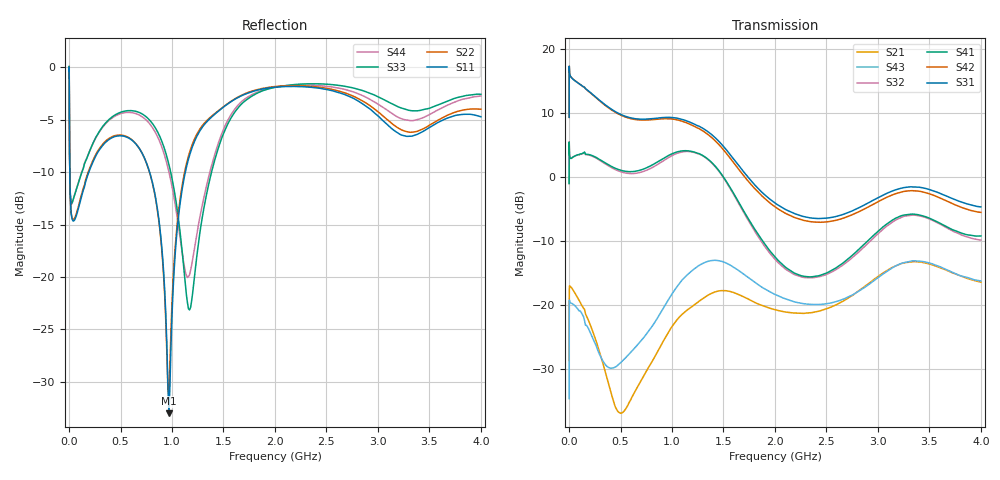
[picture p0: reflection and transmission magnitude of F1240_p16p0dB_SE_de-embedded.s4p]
! Integrated Device Technology
! Corporate Headquarters
! 6024 Silver Creek Valley Road
! San Jose, CA 95138  USA
! Phone:  1-408-284-8200
! Toll Free:  1-800-223-1366
! Webpage:  http://www.idt.com/
! Timing and RF Division
! 515 Groton Road, Suite 102
! Westford, MA 01886-6024
! Device:  F1240
! Description: Dual Intermediate Frequency Digital Variable Gain Amplifier
! Frequency:  10.0 -  500.00 MHz
! Package:  5x5 mm QFN Plastic Package: 32 pin
! Ports:  8 RF, 20 DC
!  Pin  1  = GA3 / Data  Pin 17  = RF OUT_B+
!  Pin  2  = GA4 / CLK  Pin 18  = RF OUT_B-
!  Pin  3  = GA5  Pin 19  = STBY_B
!  Pin  4  = VMODE  Pin 20  = Ground
!  Pin  5  = No Connect  Pin 21  = Ground
!  Pin  6  = GB5  Pin 22  = STB_A
!  Pin  7  = GB4  Pin 23  = RF OUT_A-  = Port 4
!  Pin  8  = GB3  Pin 24  = RF OUT_A+  = Port 3
!  Pin  9  = GB2  Pin 25  = GA0
!  Pin 10  = GB1  Pin 26  = ISET_A
!  Pin 11  = RF IN_B+  Pin 27  = VCC
!  Pin 12  = RF IN_B-  Pin 28  = Ground
!  Pin 13  = Ground  Pin 29  = RF IN_A-  = Port 2
!  Pin 14  = VCC  Pin 30  = RF IN_A+  = Port 1
!  Pin 15  = ISET_B  Pin 31  = GA1
!  Pin 16  = GB0  Pin 32  = GA2 / CSb
! Gain  = +19.5 dB
! State  = 1
! Voltage  = +5.00 V
! Current  = 85.292 mA (one channel only)
! Temperture  =  +25 C
! Test Date  =  2017-10-18
! Board  =  EB4031
! Data:  The device was measured on a custom evaluation board which has
!  individual transmission lines to the RF pins.  Data was collected
!  using a calibrated network analyzer.  The evaluation board was
!  de-embedded using Automatic Fixture Removal.
!  The reference plane is the edge of the package pin.
!  Only Channel A was measured.
!  This data is in single-ended operation.  If your needs are balanced
!  or differential S-parameters then this file needs to be used a
!  linear simulator.
! File Date:  2017-11-10  MJV
! Note:
!  Integrated Device Technology supplies this data as a sample of measured
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# Hz S dB R 100
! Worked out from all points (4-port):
!   410 points, 500 kHz to 4 GHz, reference 100 ohm
!   strongest paths, dB at 500 kHz, 930 MHz, 1.96 GHz, 2.98 GHz, 4 GHz:
!     S31: 9.3, 9.3, -3.6, -3.4, -4.7
!     S42: 9.3, 9.1, -4.2, -4.1, -5.5
!     S41: -1.0, 3.0, -11.7, -8.8, -9.2
!     S32: -1.0, 2.7, -12.1, -9.2, -9.8
!     S43: -34.6, -20.1, -18.0, -16.0, -16.2
!     S21: -28.7, -25.2, -20.5, -15.8, -16.4
!   lowest |S11| = -33.0 dB at 970 MHz (marker M1), VSWR 1.05, Z = 104 + j2.07 ohm
!   |S11| at or under -10 dB: 7.325 MHz to 191.9 MHz (184.6 MHz wide, 185 % of centre); 782.6 MHz to 1.129 GHz (346.5 MHz wide, 36.3 % of centre)
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500000  -0.34 -6.3  -28.64 8.2  -27.42 74.8  -61.34 63.1
        -28.69 7.8  -0.33 -6.2  -61.05 63.1  -27.42 75.9
        9.30 -105.3  -1.03 72.3  -0.44 1.0  -34.61 -158.3
        -1.04 73.4  9.28 -104.2  -34.59 -158.3  -0.45 3.3
3000000  -4.75 -51.8  -17.27 17.8  -19.66 12.9  -40.28 55.7
         -17.28 17.8  -4.72 -51.8  -40.22 55.5  -19.67 13.0
         16.89 -170.6  4.03 -2.4  -4.37 -47.0  -19.23 36.4
         4.03 -2.3  16.89 -170.4  -19.21 36.3  -4.43 -46.8
2.1e8  -9.53 -114.6  -23.19 -108.3  -22.59 -53.8  -33.57 8.6
       -23.25 -107.0  -9.38 -116.3  -33.57 9.0  -22.61 -53.7
       13.13 106.1  3.32 -57.7  -7.74 -81.8  -23.84 -121.2
       3.40 -57.7  13.07 105.3  -24.43 -119.8  -7.75 -81.2
5.6e8  -6.65 -174.9  -35.20 62.1  -24.28 -110.2  -27.65 -61.7
       -35.93 53.3  -6.60 -176.2  -27.81 -60.3  -24.45 -110.5
       9.38 20.4  0.57 -136.8  -4.14 -153.1  -28.48 66.5
       0.84 -138.0  9.26 19.2  -28.03 46.0  -4.30 -152.8
9.7e8  -33.01 26.4  -22.40 -46.3  -21.53 165.9  -23.06 -158.7
       -24.09 -52.5  -31.50 8.6  -23.41 -154.1  -21.98 165.3
       9.29 -79.1  3.05 134.4  -9.28 144.8  -19.11 -28.1
       3.37 129.7  9.07 -81.0  -19.03 -47.9  -9.98 148.9
1.51e9  -3.71 -143.5  -17.59 160.8  -27.64 39.0  -25.00 69.8
        -17.74 165.7  -3.68 -144.1  -24.94 75.6  -29.02 36.7
        4.56 122.5  -0.38 -46.6  -6.08 -123.3  -13.33 155.4
        -0.27 -51.6  4.02 121.1  -13.33 148.7  -5.68 -127.1
4e9  -4.71 -157.2  -16.46 58.5  -21.74 -39.7  -19.48 -48.2
     -16.43 57.8  -3.99 -150.9  -21.98 -29.7  -25.41 -24.4
     -4.69 5.0  -9.85 -126.6  -2.57 -136.2  -15.09 90.8
     -9.22 -137.1  -5.54 14.2  -16.23 63.8  -2.73 -141.4
